| IBIS file stm32l0_51_52_53_62_63_wlcsp36.ibs
| Created by s2ibis version 1.1 (customized version)
| North Carolina State University, ERL, 2006
[IBIS ver] 4.2
[File name] stm32l0_51_52_53_62_63_wlcsp36.ibs
[File Rev] 1.0
[Date]  15-10-2014
[Source] Data Created at STMicroelectronics
[Notes]  File originated from ELDO simulations.
[Disclaimer]  This information is for modeling purpose only and is
   not guaranted. The information is subject to change without
   notice.
[Copyright] Copyright 2016 STMicroelectronics Inc.
|   Component stm32l0_51_52_53_62_63_wlcsp36
[Component] stm32l0_51_52_53_62_63_wlcsp36
[Manufacturer] STMicroelectronics
[Package]
| variable   typ   min   max
R_pkg   0.0   0.0   0.0
L_pkg   0.0H   0.0H   0.0H
C_pkg   0.0F   0.0F   0.0F
[Pin]  signal_name   model_name   R_pin   L_pin   C_pin
A6 PC14-OSC32_IN io8p_wsudq_ls_ft_v33
B6 PC15-OSC32_OUT io8p_sudq_ls_tc_esdft
C6 NRST ioreset_tc_v33_esdft
E6 VREF+ POWER
D5 VDDA POWER
D4 PA0 io8p_wsudq_ls_ft_v33
F6 PA1 io8p_wsudq_lcd4_ls_ft
E5 PA2 io8p_wsudq_lcd4_ls_ft
F5 PA3 io8p_wsudq_lcd4_ls_ft
E4 PA4 io8p_wsudq_i2cin_ls_ft
F4 PA5 io8p_wsudq_i2cin_ls_ft
E3 PA6 io8p_wsudq_lcd4_ls_ft
F3 PA7 io8p_wsudq_lcd4_ls_ft
D3 PB0 io8p_wsudq_lcd4_ls_ft
C3 PB1 io8p_wsudq_lcd4_ls_ft
F2 PB2 io8p_wsudq_lcd4_ls_ft
E2 PB10 io8p_sudq_lcd4_i2cin_ls_ft
D2 PB11 io8p_sudq_lcd4_i2cin_ls_ft
F1 VDD POWER
E1 PA8 io8p_wsudq_lcd4_ls_ft
D1 PA9 io8p_wsudq_lcd4_ls_ft
C1 PA10 io8p_wsudq_lcd4_ls_ft
C2 PA11 io8usb_ls_ft
B1 PA12 io8usb_ls_ft
A1 PA13 io8p_sudq_ls_ft
B2 PA14 io8p_sudq_ls_ft
A2 PA15 io8p_wsudq_lcd4_ls_ft
B3 PB3 io8p_wsudq_lcd4_ls_ft
A3 PB4 io8p_wsudq_lcd4_ls_ft
C4 PB5 io8p_wsudq_lcd4_ls_ft
B4 PB6 io8p_wsudq_i2cin_ls_ft
A4 PB7 io8p_wsudq_i2cin_ls_ft
C5 BOOT0 vpp_test_hv
B5 PB8 io8p_sudq_lcd4_i2cin_ls_ft
D6 VSS GND
A5 VDD POWER
[Model Selector] io8p_sudq_ls_ft
io8p00_sudq_ls_ft_pd_lv  "SPEED00 1P8V, PD=40kOhm"
io8p00_sudq_ls_ft_pu_lv  "SPEED00 1P8V, PU=40kOhm"
io8p00_sudq_ls_ft_lv  "SPEED00 1P8V"
io8p01_sudq_ls_ft_pd_lv  "SPEED01 1P8V, PD=40kOhm"
io8p01_sudq_ls_ft_pu_lv  "SPEED01 1P8V, PU=40kOhm"
io8p01_sudq_ls_ft_lv  "SPEED01 1P8V"
io8p10_sudq_ls_ft_pd_lv  "SPEED10 1P8V, PD=40kOhm"
io8p10_sudq_ls_ft_pu_lv  "SPEED10 1P8V, PU=40kOhm"
io8p10_sudq_ls_ft_lv  "SPEED10 1P8V"
io8p11_sudq_ls_ft_pd_lv  "SPEED11 1P8V, PD=40kOhm"
io8p11_sudq_ls_ft_pu_lv  "SPEED11 1P8V, PU=40kOhm"
io8p11_sudq_ls_ft_lv  "SPEED11 1P8V"
io8p00_sudq_ls_ft_pd  "SPEED00, PD=40kOhm"
io8p00_sudq_ls_ft_pu  "SPEED00, PU=40kOhm"
io8p00_sudq_ls_ft  "SPEED00"
io8p01_sudq_ls_ft_pd  "SPEED01, PD=40kOhm"
io8p01_sudq_ls_ft_pu  "SPEED01, PU=40kOhm"
io8p01_sudq_ls_ft  "SPEED01"
io8p10_sudq_ls_ft_pd  "SPEED10, PD=40kOhm"
io8p10_sudq_ls_ft_pu  "SPEED10, PU=40kOhm"
io8p10_sudq_ls_ft  "SPEED10"
io8p11_sudq_ls_ft_pd  "SPEED11, PD=40kOhm"
io8p11_sudq_ls_ft_pu  "SPEED11, PU=40kOhm"
io8p11_sudq_ls_ft  "SPEED11"
[Model Selector] io8p_sudq_ls_tc_esdft
io8p00_sudq_ls_tc_esdft_pd_lv  "SPEED00 1P8V, PD=40kOhm"
io8p00_sudq_ls_tc_esdft_pu_lv  "SPEED00 1P8V, PU=40kOhm"
io8p00_sudq_ls_tc_esdft_lv  "SPEED00 1P8V"
io8p01_sudq_ls_tc_esdft_pd_lv  "SPEED01 1P8V, PD=40kOhm"
io8p01_sudq_ls_tc_esdft_pu_lv  "SPEED01 1P8V, PU=40kOhm"
io8p01_sudq_ls_tc_esdft_lv  "SPEED01 1P8V"
io8p10_sudq_ls_tc_esdft_pd_lv  "SPEED10 1P8V, PD=40kOhm"
io8p10_sudq_ls_tc_esdft_pu_lv  "SPEED10 1P8V, PU=40kOhm"
io8p10_sudq_ls_tc_esdft_lv  "SPEED10 1P8V"
io8p11_sudq_ls_tc_esdft_pd_lv  "SPEED11 1P8V, PD=40kOhm"
io8p11_sudq_ls_tc_esdft_pu_lv  "SPEED11 1P8V, PU=40kOhm"
io8p11_sudq_ls_tc_esdft_lv  "SPEED11 1P8V"
io8p00_sudq_ls_tc_esdft_pd  "SPEED00, PD=40kOhm"
io8p00_sudq_ls_tc_esdft_pu  "SPEED00, PU=40kOhm"
io8p00_sudq_ls_tc_esdft  "SPEED00"
io8p01_sudq_ls_tc_esdft_pd  "SPEED01, PD=40kOhm"
io8p01_sudq_ls_tc_esdft_pu  "SPEED01, PU=40kOhm"
io8p01_sudq_ls_tc_esdft  "SPEED01"
io8p10_sudq_ls_tc_esdft_pd  "SPEED10, PD=40kOhm"
io8p10_sudq_ls_tc_esdft_pu  "SPEED10, PU=40kOhm"
io8p10_sudq_ls_tc_esdft  "SPEED10"
io8p11_sudq_ls_tc_esdft_pd  "SPEED11, PD=40kOhm"
io8p11_sudq_ls_tc_esdft_pu  "SPEED11, PU=40kOhm"
io8p11_sudq_ls_tc_esdft  "SPEED11"
[Model Selector] io8p_wsudq_i2cin_ls_ft
io8p00_wsudq_i2cin_ls_ft_pd_lv  "SPEED00 1P8V, PD=40kOhm"
io8p00_wsudq_i2cin_ls_ft_pu_lv  "SPEED00 1P8V, PU=40kOhm"
io8p00_wsudq_i2cin_ls_ft_lv  "SPEED00 1P8V"
io8p01_wsudq_i2cin_ls_ft_pd_lv  "SPEED01 1P8V, PD=40kOhm"
io8p01_wsudq_i2cin_ls_ft_pu_lv  "SPEED01 1P8V, PU=40kOhm"
io8p01_wsudq_i2cin_ls_ft_lv  "SPEED01 1P8V"
io8p10_wsudq_i2cin_ls_ft_pd_lv  "SPEED10 1P8V, PD=40kOhm"
io8p10_wsudq_i2cin_ls_ft_pu_lv  "SPEED10 1P8V, PU=40kOhm"
io8p10_wsudq_i2cin_ls_ft_lv  "SPEED10 1P8V"
io8p11_wsudq_i2cin_ls_ft_pd_lv  "SPEED11 1P8V, PD=40kOhm"
io8p11_wsudq_i2cin_ls_ft_pu_lv  "SPEED11 1P8V, PU=40kOhm"
io8p11_wsudq_i2cin_ls_ft_lv  "SPEED11 1P8V"
io8p00_wsudq_i2cin_ls_ft_pd  "SPEED00, PD=40kOhm"
io8p00_wsudq_i2cin_ls_ft_pu  "SPEED00, PU=40kOhm"
io8p00_wsudq_i2cin_ls_ft  "SPEED00"
io8p01_wsudq_i2cin_ls_ft_pd  "SPEED01, PD=40kOhm"
io8p01_wsudq_i2cin_ls_ft_pu  "SPEED01, PU=40kOhm"
io8p01_wsudq_i2cin_ls_ft  "SPEED01"
io8p10_wsudq_i2cin_ls_ft_pd  "SPEED10, PD=40kOhm"
io8p10_wsudq_i2cin_ls_ft_pu  "SPEED10, PU=40kOhm"
io8p10_wsudq_i2cin_ls_ft  "SPEED10"
io8p11_wsudq_i2cin_ls_ft_pd  "SPEED11, PD=40kOhm"
io8p11_wsudq_i2cin_ls_ft_pu  "SPEED11, PU=40kOhm"
io8p11_wsudq_i2cin_ls_ft  "SPEED11"
[Model Selector] io8p_wsudq_lcd4_ls_ft
io8p00_wsudq_lcd4_ls_ft_pd_lv  "SPEED00 1P8V, PD=40kOhm"
io8p00_wsudq_lcd4_ls_ft_pu_lv  "SPEED00 1P8V, PU=40kOhm"
io8p00_wsudq_lcd4_ls_ft_lv  "SPEED00 1P8V"
io8p01_wsudq_lcd4_ls_ft_pd_lv  "SPEED01 1P8V, PD=40kOhm"
io8p01_wsudq_lcd4_ls_ft_pu_lv  "SPEED01 1P8V, PU=40kOhm"
io8p01_wsudq_lcd4_ls_ft_lv  "SPEED01 1P8V"
io8p10_wsudq_lcd4_ls_ft_pd_lv  "SPEED10 1P8V, PD=40kOhm"
io8p10_wsudq_lcd4_ls_ft_pu_lv  "SPEED10 1P8V, PU=40kOhm"
io8p10_wsudq_lcd4_ls_ft_lv  "SPEED10 1P8V"
io8p11_wsudq_lcd4_ls_ft_pd_lv  "SPEED11 1P8V, PD=40kOhm"
io8p11_wsudq_lcd4_ls_ft_pu_lv  "SPEED11 1P8V, PU=40kOhm"
io8p11_wsudq_lcd4_ls_ft_lv  "SPEED11 1P8V"
io8p00_wsudq_lcd4_ls_ft_pd  "SPEED00, PD=40kOhm"
io8p00_wsudq_lcd4_ls_ft_pu  "SPEED00, PU=40kOhm"
io8p00_wsudq_lcd4_ls_ft  "SPEED00"
io8p01_wsudq_lcd4_ls_ft_pd  "SPEED01, PD=40kOhm"
io8p01_wsudq_lcd4_ls_ft_pu  "SPEED01, PU=40kOhm"
io8p01_wsudq_lcd4_ls_ft  "SPEED01"
io8p10_wsudq_lcd4_ls_ft_pd  "SPEED10, PD=40kOhm"
io8p10_wsudq_lcd4_ls_ft_pu  "SPEED10, PU=40kOhm"
io8p10_wsudq_lcd4_ls_ft  "SPEED10"
io8p11_wsudq_lcd4_ls_ft_pd  "SPEED11, PD=40kOhm"
io8p11_wsudq_lcd4_ls_ft_pu  "SPEED11, PU=40kOhm"
io8p11_wsudq_lcd4_ls_ft  "SPEED11"
[Model Selector] io8p_wsudq_ls_ft_v33
io8p00_wsudq_ls_ft_v33_pd_lv  "SPEED00 1P8V, PD=40kOhm"
io8p00_wsudq_ls_ft_v33_pu_lv  "SPEED00 1P8V, PU=40kOhm"
io8p00_wsudq_ls_ft_v33_lv  "SPEED00 1P8V"
io8p01_wsudq_ls_ft_v33_pd_lv  "SPEED01 1P8V, PD=40kOhm"
io8p01_wsudq_ls_ft_v33_pu_lv  "SPEED01 1P8V, PU=40kOhm"
io8p01_wsudq_ls_ft_v33_lv  "SPEED01 1P8V"
io8p10_wsudq_ls_ft_v33_pd_lv  "SPEED10 1P8V, PD=40kOhm"
io8p10_wsudq_ls_ft_v33_pu_lv  "SPEED10 1P8V, PU=40kOhm"
io8p10_wsudq_ls_ft_v33_lv  "SPEED10 1P8V"
io8p11_wsudq_ls_ft_v33_pd_lv  "SPEED11 1P8V, PD=40kOhm"
io8p11_wsudq_ls_ft_v33_pu_lv  "SPEED11 1P8V, PU=40kOhm"
io8p11_wsudq_ls_ft_v33_lv  "SPEED11 1P8V"
io8p00_wsudq_ls_ft_v33_pd  "SPEED00, PD=40kOhm"
io8p00_wsudq_ls_ft_v33_pu  "SPEED00, PU=40kOhm"
io8p00_wsudq_ls_ft_v33  "SPEED00"
io8p01_wsudq_ls_ft_v33_pd  "SPEED01, PD=40kOhm"
io8p01_wsudq_ls_ft_v33_pu  "SPEED01, PU=40kOhm"
io8p01_wsudq_ls_ft_v33  "SPEED01"
io8p10_wsudq_ls_ft_v33_pd  "SPEED10, PD=40kOhm"
io8p10_wsudq_ls_ft_v33_pu  "SPEED10, PU=40kOhm"
io8p10_wsudq_ls_ft_v33  "SPEED10"
io8p11_wsudq_ls_ft_v33_pd  "SPEED11, PD=40kOhm"
io8p11_wsudq_ls_ft_v33_pu  "SPEED11, PU=40kOhm"
io8p11_wsudq_ls_ft_v33  "SPEED11"
[Model Selector] ioreset_tc_v33_esdft
ioreset_tc_v33_esdft_pu_lv  "IORESET 1P65V + PU=40kOhm"
ioreset_tc_v33_esdft_nopu_lv  "IORESET 1P65V"
ioreset_tc_v33_esdft_pu  "IORESET + PU=40kOhm"
ioreset_tc_v33_esdft_nopu  "IORESET"
[Model Selector] vpp_test_hv
vpp_test_hv_2p4  "Input Buffer 1P65V"
vpp_test_hv_3p3  "Input Buffer"
[Model Selector] io8usb_ls_ft
io8usb_ls_ft_dpdn_pu  "HS USB DP/DN IO + PU=1.2kOhm"
io8usb_ls_ft_dpdn  "HS USB DP/DN IO"
io8p00_ls_ft_pd_lv  "SPEED00 1P8V, PD=40kOhm"
io8p00_ls_ft_pu_lv  "SPEED00 1P8V, PU=40kOhm"
io8p00_ls_ft_lv  "SPEED00 1P8V"
io8p01_ls_ft_pd_lv  "SPEED01 1P8V, PD=40kOhm"
io8p01_ls_ft_pu_lv  "SPEED01 1P8V, PU=40kOhm"
io8p01_ls_ft_lv  "SPEED01 1P8V"
io8p10_ls_ft_pd_lv  "SPEED10 1P8V, PD=40kOhm"
io8p10_ls_ft_pu_lv  "SPEED10 1P8V, PU=40kOhm"
io8p10_ls_ft_lv  "SPEED10 1P8V"
io8p11_ls_ft_pd_lv  "SPEED11 1P8V, PD=40kOhm"
io8p11_ls_ft_pu_lv  "SPEED11 1P8V, PU=40kOhm"
io8p11_ls_ft_lv  "SPEED11 1P8V"
io8p00_ls_ft_pd  "SPEED00, PD=40kOhm"
io8p00_ls_ft_pu  "SPEED00, PU=40kOhm"
io8p00_ls_ft  "SPEED00"
io8p01_ls_ft_pd  "SPEED01, PD=40kOhm"
io8p01_ls_ft_pu  "SPEED01, PU=40kOhm"
io8p01_ls_ft  "SPEED01"
io8p10_ls_ft_pd  "SPEED10, PD=40kOhm"
io8p10_ls_ft_pu  "SPEED10, PU=40kOhm"
io8p10_ls_ft  "SPEED10"
io8p11_ls_ft_pd  "SPEED11, PD=40kOhm"
io8p11_ls_ft_pu  "SPEED11, PU=40kOhm"
io8p11_ls_ft  "SPEED11"
[Model Selector] io8p_sudq_lcd4_i2cin_ls_ft
io8p00_sudq_lcd4_i2cin_ls_ft_pd_lv  "SPEED00 1P8V, PD=40kOhm"
io8p00_sudq_lcd4_i2cin_ls_ft_pu_lv  "SPEED00 1P8V, PU=40kOhm"
io8p00_sudq_lcd4_i2cin_ls_ft_lv  "SPEED00 1P8V"
io8p01_sudq_lcd4_i2cin_ls_ft_pd_lv  "SPEED01 1P8V, PD=40kOhm"
io8p01_sudq_lcd4_i2cin_ls_ft_pu_lv  "SPEED01 1P8V, PU=40kOhm"
io8p01_sudq_lcd4_i2cin_ls_ft_lv  "SPEED01 1P8V"
io8p10_sudq_lcd4_i2cin_ls_ft_pd_lv  "SPEED10 1P8V, PD=40kOhm"
io8p10_sudq_lcd4_i2cin_ls_ft_pu_lv  "SPEED10 1P8V, PU=40kOhm"
io8p10_sudq_lcd4_i2cin_ls_ft_lv  "SPEED10 1P8V"
io8p11_sudq_lcd4_i2cin_ls_ft_pd_lv  "SPEED11 1P8V, PD=40kOhm"
io8p11_sudq_lcd4_i2cin_ls_ft_pu_lv  "SPEED11 1P8V, PU=40kOhm"
io8p11_sudq_lcd4_i2cin_ls_ft_lv  "SPEED11 1P8V"
io8p00_sudq_lcd4_i2cin_ls_ft_pd  "SPEED00, PD=40kOhm"
io8p00_sudq_lcd4_i2cin_ls_ft_pu  "SPEED00, PU=40kOhm"
io8p00_sudq_lcd4_i2cin_ls_ft  "SPEED00"
io8p01_sudq_lcd4_i2cin_ls_ft_pd  "SPEED01, PD=40kOhm"
io8p01_sudq_lcd4_i2cin_ls_ft_pu  "SPEED01, PU=40kOhm"
io8p01_sudq_lcd4_i2cin_ls_ft  "SPEED01"
io8p10_sudq_lcd4_i2cin_ls_ft_pd  "SPEED10, PD=40kOhm"
io8p10_sudq_lcd4_i2cin_ls_ft_pu  "SPEED10, PU=40kOhm"
io8p10_sudq_lcd4_i2cin_ls_ft  "SPEED10"
io8p11_sudq_lcd4_i2cin_ls_ft_pd  "SPEED11, PD=40kOhm"
io8p11_sudq_lcd4_i2cin_ls_ft_pu  "SPEED11, PU=40kOhm"
io8p11_sudq_lcd4_i2cin_ls_ft  "SPEED11"
| Models and submodels in the file (176): io8p00_sudq_ls_ft_pd_lv (I/O), io8p00_sudq_ls_ft_pu_lv (I/O), io8p00_sudq_ls_ft_lv (I/O), io8p01_sudq_ls_ft_pd_lv (I/O), io8p01_sudq_ls_ft_pu_lv (I/O), io8p01_sudq_ls_ft_lv (I/O), io8p10_sudq_ls_ft_pd_lv (I/O), io8p10_sudq_ls_ft_pu_lv (I/O), io8p10_sudq_ls_ft_lv (I/O), io8p11_sudq_ls_ft_pd_lv (I/O), io8p11_sudq_ls_ft_pu_lv (I/O), io8p11_sudq_ls_ft_lv (I/O), io8p00_sudq_ls_ft_pd (I/O), io8p00_sudq_ls_ft_pu (I/O), io8p00_sudq_ls_ft (I/O), io8p01_sudq_ls_ft_pd (I/O), io8p01_sudq_ls_ft_pu (I/O), io8p01_sudq_ls_ft (I/O), io8p10_sudq_ls_ft_pd (I/O), io8p10_sudq_ls_ft_pu (I/O), io8p10_sudq_ls_ft (I/O), io8p11_sudq_ls_ft_pd (I/O), io8p11_sudq_ls_ft_pu (I/O), io8p11_sudq_ls_ft (I/O), io8p00_sudq_ls_tc_esdft_pd_lv (I/O), io8p00_sudq_ls_tc_esdft_pu_lv (I/O), io8p00_sudq_ls_tc_esdft_lv (I/O), io8p01_sudq_ls_tc_esdft_pd_lv (I/O), io8p01_sudq_ls_tc_esdft_pu_lv (I/O), io8p01_sudq_ls_tc_esdft_lv (I/O), io8p10_sudq_ls_tc_esdft_pd_lv (I/O), io8p10_sudq_ls_tc_esdft_pu_lv (I/O), io8p10_sudq_ls_tc_esdft_lv (I/O), io8p11_sudq_ls_tc_esdft_pd_lv (I/O), io8p11_sudq_ls_tc_esdft_pu_lv (I/O), io8p11_sudq_ls_tc_esdft_lv (I/O), io8p00_sudq_ls_tc_esdft_pd (I/O), io8p00_sudq_ls_tc_esdft_pu (I/O), io8p00_sudq_ls_tc_esdft (I/O), io8p01_sudq_ls_tc_esdft_pd (I/O), io8p01_sudq_ls_tc_esdft_pu (I/O), io8p01_sudq_ls_tc_esdft (I/O), io8p10_sudq_ls_tc_esdft_pd (I/O), io8p10_sudq_ls_tc_esdft_pu (I/O), io8p10_sudq_ls_tc_esdft (I/O), io8p11_sudq_ls_tc_esdft_pd (I/O), io8p11_sudq_ls_tc_esdft_pu (I/O), io8p11_sudq_ls_tc_esdft (I/O), io8p00_wsudq_i2cin_ls_ft_pd_lv (I/O), io8p00_wsudq_i2cin_ls_ft_pu_lv (I/O), io8p00_wsudq_i2cin_ls_ft_lv (I/O), io8p01_wsudq_i2cin_ls_ft_pd_lv (I/O), io8p01_wsudq_i2cin_ls_ft_pu_lv (I/O), io8p01_wsudq_i2cin_ls_ft_lv (I/O), io8p10_wsudq_i2cin_ls_ft_pd_lv (I/O), io8p10_wsudq_i2cin_ls_ft_pu_lv (I/O), io8p10_wsudq_i2cin_ls_ft_lv (I/O), io8p11_wsudq_i2cin_ls_ft_pd_lv (I/O), io8p11_wsudq_i2cin_ls_ft_pu_lv (I/O), io8p11_wsudq_i2cin_ls_ft_lv (I/O), io8p00_wsudq_i2cin_ls_ft_pd (I/O), io8p00_wsudq_i2cin_ls_ft_pu (I/O), io8p00_wsudq_i2cin_ls_ft (I/O), io8p01_wsudq_i2cin_ls_ft_pd (I/O), io8p01_wsudq_i2cin_ls_ft_pu (I/O), io8p01_wsudq_i2cin_ls_ft (I/O), io8p10_wsudq_i2cin_ls_ft_pd (I/O), io8p10_wsudq_i2cin_ls_ft_pu (I/O), io8p10_wsudq_i2cin_ls_ft (I/O), io8p11_wsudq_i2cin_ls_ft_pd (I/O), io8p11_wsudq_i2cin_ls_ft_pu (I/O), io8p11_wsudq_i2cin_ls_ft (I/O), io8p00_wsudq_lcd4_ls_ft_pd_lv (I/O), io8p00_wsudq_lcd4_ls_ft_pu_lv (I/O), io8p00_wsudq_lcd4_ls_ft_lv (I/O), io8p01_wsudq_lcd4_ls_ft_pd_lv (I/O), io8p01_wsudq_lcd4_ls_ft_pu_lv (I/O), io8p01_wsudq_lcd4_ls_ft_lv (I/O), io8p10_wsudq_lcd4_ls_ft_pd_lv (I/O), io8p10_wsudq_lcd4_ls_ft_pu_lv (I/O)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
